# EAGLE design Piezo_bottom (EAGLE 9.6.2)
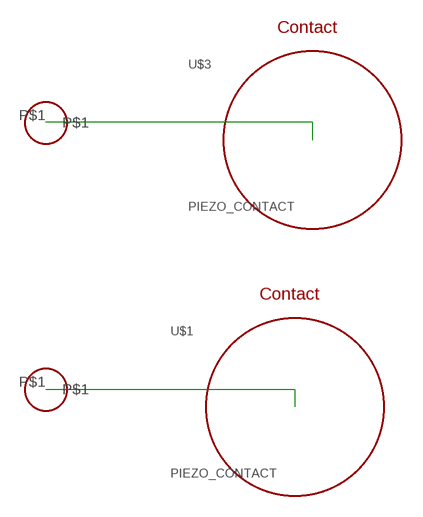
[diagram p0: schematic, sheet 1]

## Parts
U$1  PIEZO_CONTACT  [PIEZO_CONTACT]
U$2  SPRING_PADSINGLE_SIDE  [SPRINGPAD_SINGLE_SIDE]
U$3  PIEZO_CONTACT  [PIEZO_CONTACT]
U$4  SPRING_PAD  [SPRING_PAD]

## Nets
N$1 [connect]: U$1.P$1 U$2.P$1
N$2 [connect]: U$3.P$1 U$4.P$1

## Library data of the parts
U$1 U$3 = RGB_library:PIEZO_CONTACT
U$2 U$4 = RGB_library:SPRING_PAD

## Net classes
1 connect: width 1.016 mm, clearance 0.152 mm

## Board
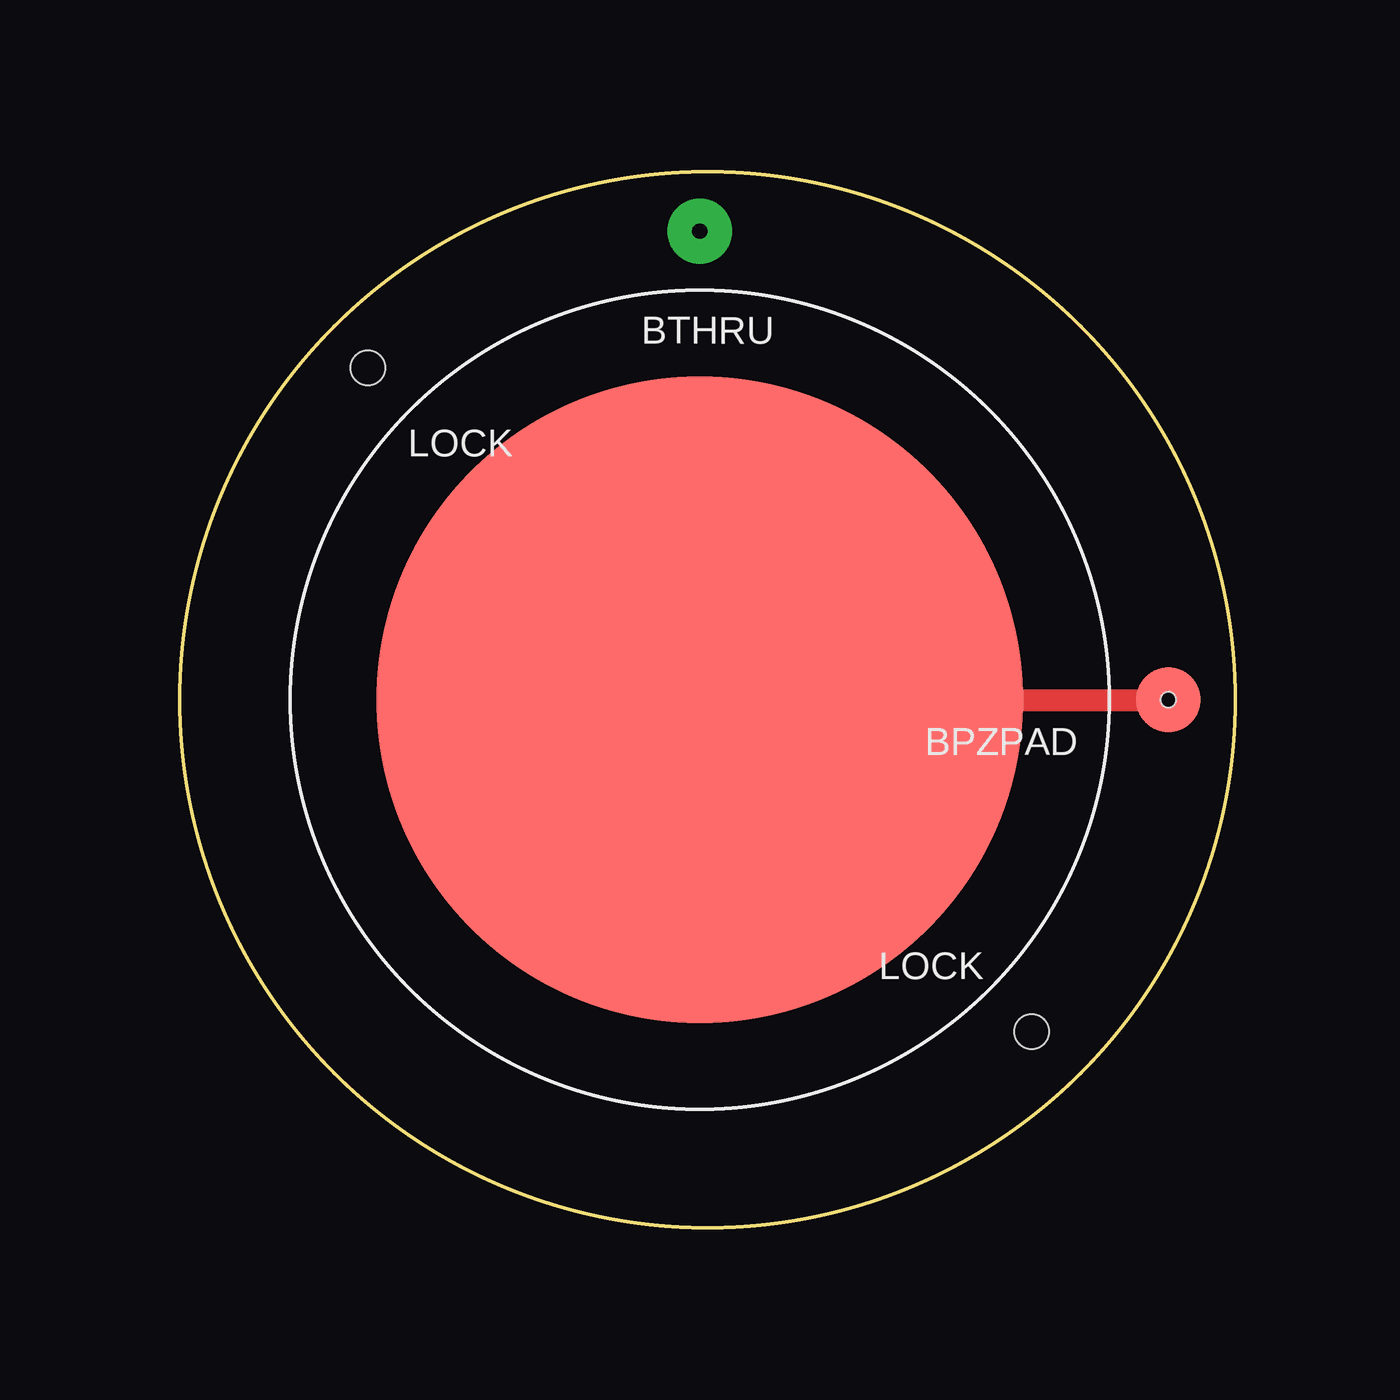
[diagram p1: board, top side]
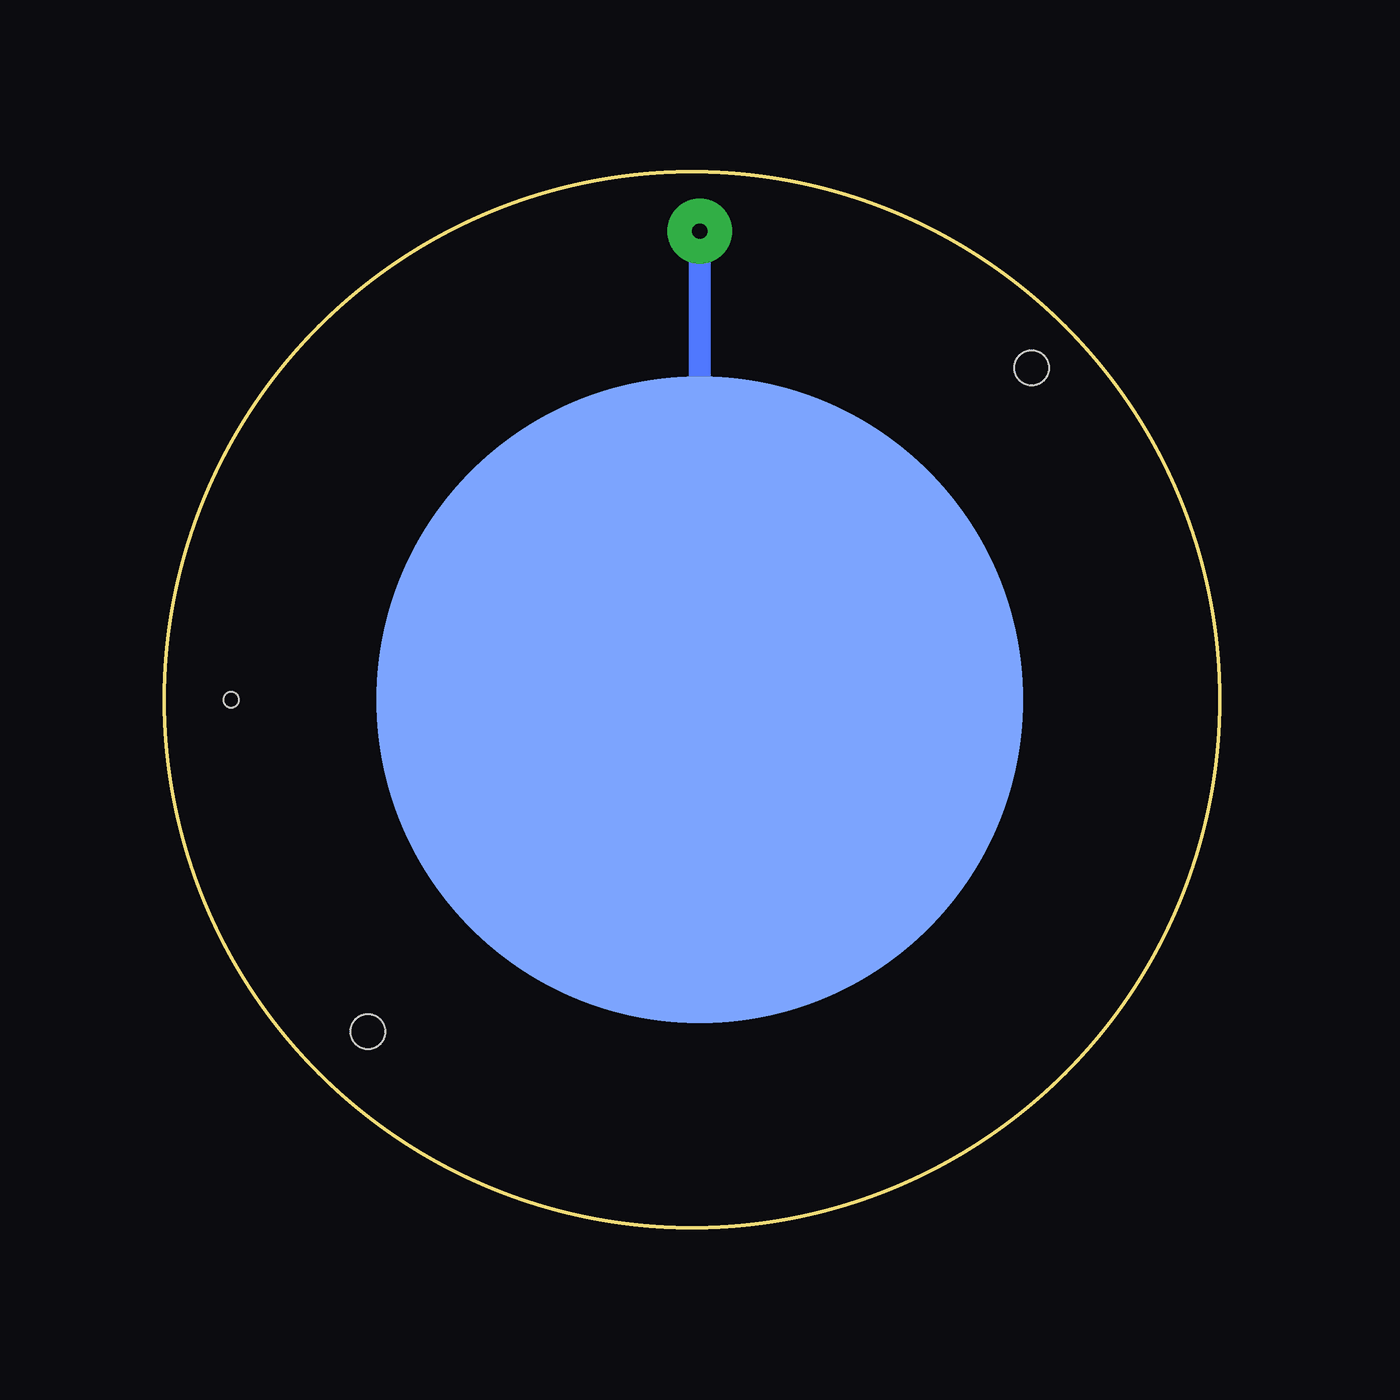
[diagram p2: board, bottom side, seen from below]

Size 49 x 49 mm. Coordinates in mm from the lower left corner, seen from the top.
Outline: circle at 24.5,24.5 radius 24.5
Copper layers (1*16): Top 0.035mm / dielectric 1.5mm / Bottom 0.035mm
Design rules "default": minimum track width 6mil, minimum drill 0.35mm, track to track 6mil, track to pad 6mil, pad to pad 6mil, via to via 6mil, smd to smd 6mil, copper to edge 40mil, drill to drill 6mil, minimum pad ring 10mil, minimum via ring 8mil, stop-mask expansion 4mil, vias tented up to drill 0mil, thermal gap 10mil
Holes 1.6 mm at 8.74,39.9 39.54,9.1

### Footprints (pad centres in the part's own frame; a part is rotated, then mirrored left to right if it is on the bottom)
PIEZO_CONTACT = smd 30 x 30: P$1 0,0
SPRINGPAD_SINGLE_SIDE = smd 3 x 3: P$1 0,0 | hole 0.7: 0,0
SPRING_PAD = drill 0.7 pad 3: P$1 0,0

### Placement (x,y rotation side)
U$1  24.14,24.5 0 top
U$2  45.89,24.5 0 top
U$3  24.14,24.5 0 bottom
U$4  24.14,46.25 0 top

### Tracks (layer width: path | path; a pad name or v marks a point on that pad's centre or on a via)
N$1
  Top 1.016: U$1.P$1 U$2.P$1
N$2
  Bottom 1.016: U$3.P$1 U$4.P$1

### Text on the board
tNames: BTHRU | LOCK | BPZPAD | LOCK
